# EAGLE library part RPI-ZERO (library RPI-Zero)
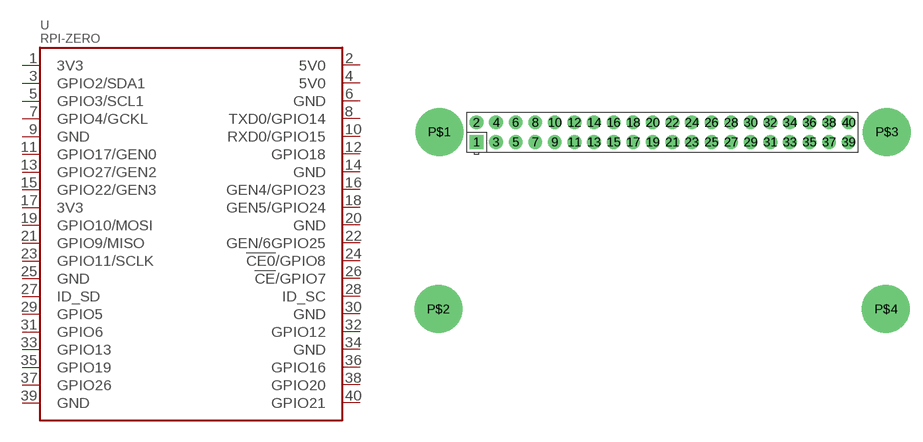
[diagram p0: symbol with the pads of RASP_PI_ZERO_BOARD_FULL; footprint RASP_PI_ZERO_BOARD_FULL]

Designator prefix -

## RPI-ZERO  [RASP_PI_ZERO_BOARD_FULL]
1  3V3  sup
2  5V0  sup
3  GPIO2/SDA1
4  5V0  sup
5  GPIO3/SCL1
6  GND  sup
7  GPIO4/GCKL
8  TXD0/GPIO14
9  GND  sup
10  RXD0/GPIO15
11  GPIO17/GEN0
12  GPIO18
13  GPIO27/GEN2
14  GND  sup
15  GPIO22/GEN3
16  GEN4/GPIO23
17  3V3  sup
18  GEN5/GPIO24
19  GPIO10/MOSI
20  GND  sup
21  GPIO9/MISO
22  GEN/6GPIO25
23  GPIO11/SCLK
24  !CE0!/GPIO8
25  GND  sup
26  !CE!/GPIO7
27  ID_SD
28  ID_SC
29  GPIO5
30  GND  sup
31  GPIO6
32  GPIO12
33  GPIO13
34  GND  sup
35  GPIO19
36  GPIO16
37  GPIO26
38  GPIO20
39  GND  sup
40  GPIO21

## Footprint RASP_PI_ZERO_BOARD_FULL (pad centres in mm)
Raspberry Pi board model B+, full outline with position of big connectors & drill holes
drill 1 pad 1.778 square: 1 10.148,25.357
drill 1 pad 1.778: 2 10.148,27.897; 3 12.688,25.357; 4 12.688,27.897; 5 15.228,25.357; 6 15.228,27.897; 7 17.768,25.357; 8 17.768,27.897; 9 20.308,25.357; 10 20.308,27.897; 11 22.848,25.357; 12 22.848,27.897; 13 25.388,25.357; 14 25.388,27.897; 15 27.928,25.357; 16 27.928,27.897; 17 30.468,25.357; 18 30.468,27.897; 19 33.008,25.357; 20 33.008,27.897; 21 35.548,25.357; 22 35.548,27.897; 23 38.088,25.357; 24 38.088,27.897; 25 40.628,25.357; 26 40.628,27.897; 27 43.168,25.357; 28 43.168,27.897; 29 45.708,25.357; 30 45.708,27.897; 31 48.248,25.357; 32 48.248,27.897; 33 50.788,25.357; 34 50.788,27.897; 35 53.328,25.357; 36 53.328,27.897; 37 55.868,25.357; 38 55.868,27.897; 39 58.408,25.357; 40 58.408,27.897
drill 3.048 pad 6.223: P$1 5.334,26.67; P$2 5.207,3.683; P$3 63.373,26.67; P$4 63.246,3.683

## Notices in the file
Konrad Meyer (c) 2011
